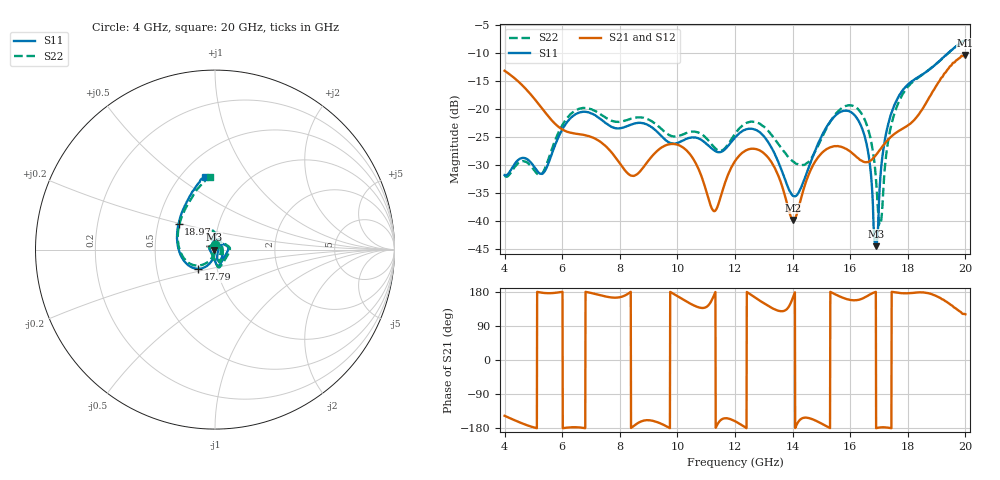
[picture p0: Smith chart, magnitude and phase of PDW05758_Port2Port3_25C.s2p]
! "!Agilent Technologies,E8361A,US43140610,A.07.50.67"
!Agilent E8361A: A.07.50.67
! "!Date: Friday, February 28, 2014 12:27:08"
! "!Correction: S11(Full 2 Port(1,2)) "
! "!S21(Full 2 Port(1,2)) "
! "!S12(Full 2 Port(1,2)) "
! "!S22(Full 2 Port(1,2)) "
! "!S2P File: Measurements: S11, S21, S12, S22:"
!Power divider measured mounted on 10mil RO4350 with coaxial edge launch connectors.  Coaxial connectors have been gated out.  Unused port was externally terminated
!with coaxial termination.  Measurement reference plane placed at the part edge.  The loss of the test board and connectors has been removed.
!Port one = one output port
!Port two = second output port
# GHz S MA R 50
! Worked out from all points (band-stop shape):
!   1601 points, 4 GHz to 20 GHz, reference 50 ohm
!   highest |S21| = -10.43 dB at 19.99 GHz (marker M1); lowest = -39.9 dB at 14.03 GHz (marker M2)
!   |S21| within 3 dB of the highest: start of sweep to 4.055 GHz; 19.33 GHz to end of sweep
!   lowest |S11| = -44.5 dB at 16.89 GHz (marker M3), VSWR 1.01, Z = 49.4 + j0.0271 ohm
!   |S11| at or under -10 dB: start of sweep to 19.42 GHz
!   |S22| runs from -40.8 to -7.8 dB; largest |S21 - S12| = 0.015
!   S11 on the Smith chart (normalised r, x): 4 GHz: 1.00, +0.05; 17.79 GHz: 0.81, -0.18; 18.97 GHz: 0.64, +0.20; 20 GHz: 0.65, +0.63
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4  0.02558 91.6  0.218 -147.2  0.2179 -147.2  0.02528 86.1
4.63  0.03641 152.3  0.1602 -167.9  0.1602 -167.9  0.03405 151.4
5.28  0.0262 -152.2  0.1021 177.7  0.1021 177.7  0.02604 -144.4
6.67  0.09333 -80.9  0.05886 -178.5  0.05869 -178.4  0.1008 -78.4
8.42  0.07254 -3.1  0.02522 -177.7  0.02522 -177.7  0.08182 -5.9
9.34  0.06068 26.0  0.04296 -165.1  0.04296 -165.1  0.06969 21.5
10.37  0.05455 77.7  0.04109 152.0  0.04105 151.9  0.06147 71.2
11.27  0.04258 35.2  0.01219 170.6  0.01219 170.8  0.04551 36.5
12  0.05523 -43.9  0.03406 -161.5  0.03414 -161.7  0.05969 -46.9
13.06  0.05436 -76.6  0.03887 147.0  0.03866 146.7  0.06689 -71.2
14.03  0.01662 0.5  0.01015 168.8  0.01013 168.6  0.03372 -15.7
14.67  0.03566 90.7  0.02992 -155.8  0.02982 -155.8  0.03684 56.4
15.48  0.08661 116.1  0.04633 173.2  0.04629 173.4  0.08862 98.3
16.19  0.08526 109.1  0.03771 157.6  0.0378 157.7  0.103 94.2
16.62  0.04123 98.7  0.03339 169.9  0.03347 170.0  0.06594 83.1
16.89  0.005932 177.3  0.03845 179.8  0.03843 179.9  0.02454 67.5
17.05  0.02501 -97.7  0.04351 -177.8  0.04354 -177.7  0.009269 -27.4
17.34  0.07618 -109.3  0.05366 -178.9  0.05364 -178.6  0.05567 -112.9
17.79  0.1425 -131.2  0.06562 176.2  0.06591 176.3  0.1304 -136.8
18.97  0.2492 144.6  0.1573 169.3  0.1579 169.5  0.2488 141.4
19.99  0.4049 98.2  0.3011 120.9  0.2903 119.1  0.4051 93.8
20  0.4061 98.0  0.3007 120.6  0.2904 118.6  0.4065 93.6
